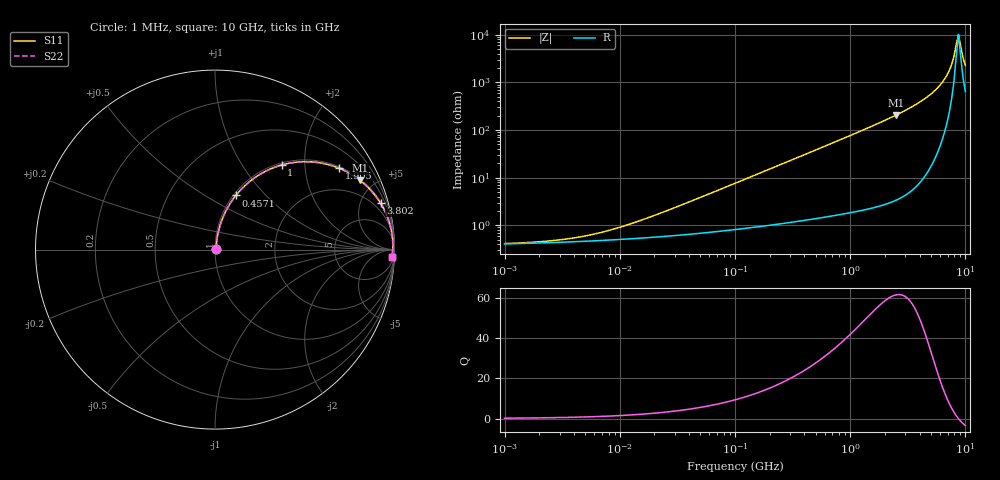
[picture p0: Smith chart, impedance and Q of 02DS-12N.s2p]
# MHz S MA R 50
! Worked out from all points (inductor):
!   201 points, 1 MHz to 10 GHz, reference 50 ohm
!   read as one part in series: L = 12 nH near 22.91 MHz
!   highest Q = 61.5 at 2.512 GHz (marker M1), where L = 13.1 nH
!   self-resonance near 8.318 GHz
!   S11 on the Smith chart (normalised r, x): 1 MHz: 1.01, +0.00; 457.1 MHz: 1.03, +0.69; 1 GHz: 1.04, +1.53; 1.905 GHz: 1.05, +3.02; 3.802 GHz: 1.13, +7.09; 10 GHz: 14, -43
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1  0.004103 10.5  0.996 -0.0  0.996 -0.0  0.004103 10.5
2.39883  0.004642 22.7  0.9957 -0.1  0.9957 -0.1  0.004642 22.7
4.7863  0.005808 38.0  0.9954 -0.2  0.9954 -0.2  0.005808 38.0
9.54993  0.008717 54.9  0.995 -0.4  0.995 -0.4  0.008717 54.9
21.8776  0.01735 70.0  0.9942 -0.9  0.9942 -0.9  0.01735 70.0
104.713  0.0785 79.6  0.9888 -4.5  0.9888 -4.5  0.0785 79.6
229.087  0.1689 76.8  0.9755 -9.7  0.9755 -9.7  0.1689 76.8
457.088  0.323 69.0  0.9341 -18.8  0.9341 -18.8  0.323 69.0
478.63  0.3366 68.2  0.9292 -19.7  0.9292 -19.7  0.3366 68.2
1000  0.6004 51.7  0.7855 -36.9  0.7855 -36.9  0.6004 51.7
1380.38  0.7227 42.6  0.6767 -46.3  0.6767 -46.3  0.7227 42.6
1905.46  0.8271 33.2  0.5479 -55.8  0.5479 -55.8  0.8271 33.2
2187.76  0.8635 29.3  0.4902 -59.7  0.4902 -59.7  0.8635 29.3
2511.89  0.8945 25.6  0.4328 -63.4  0.4328 -63.4  0.8945 25.6
3801.89  0.9577 15.7  0.2701 -73.2  0.2701 -73.2  0.9577 15.7
5248.07  0.9822 9.1  0.1577 -79.0  0.1577 -79.0  0.9822 9.1
6606.93  0.9899 4.8  0.08412 -80.7  0.08412 -80.7  0.9899 4.8
7585.78  0.9913 2.4  0.0421 -76.8  0.0421 -76.8  0.9913 2.4
7943.28  0.9912 1.6  0.02864 -71.3  0.02864 -71.3  0.9912 1.6
8709.64  0.9902 -0.0  0.009778 2.5  0.009778 2.5  0.9902 -0.0
9549.93  0.9882 -1.6  0.03034 66.3  0.03034 66.3  0.9882 -1.6
10000  0.9868 -2.4  0.04373 71.2  0.04373 71.2  0.9868 -2.4
